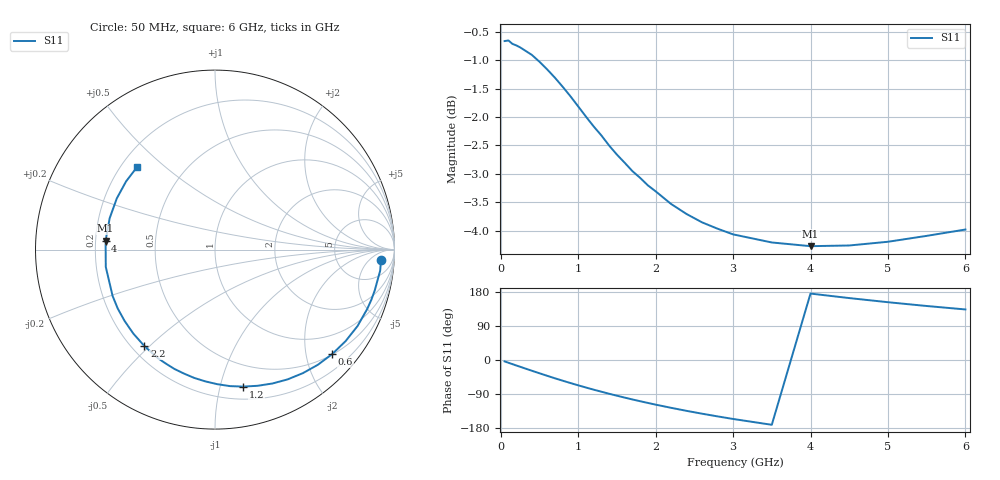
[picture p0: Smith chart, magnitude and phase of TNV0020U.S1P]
! SIEMENS Discrete & RF Semiconductors
! BAS70-07W
! Si Schottky Diode in SOT343
! IF = 0.02 mA
! S-Parameters:  February  1997
# GHz  S  MA  R  50
!  f  S11
! GHz  MAG  ANG
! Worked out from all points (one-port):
!   34 points, 50 MHz to 6 GHz, reference 50 ohm
!   lowest |S11| = -4.3 dB at 4 GHz (marker M1), VSWR 4.15, Z = 12.1 + j1.93 ohm
!   |S11| at or under -10 dB: nowhere
!   S11 on the Smith chart (normalised r, x): 50 MHz: 15, -13; 600 MHz: 0.51, -2.54; 1.2 GHz: 0.30, -1.18; 2.2 GHz: 0.25, -0.48; 4 GHz: 0.24, +0.04; 6 GHz: 0.26, +0.41
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0.05  0.9266 -3.7
0.1  0.9277 -7.3
0.15  0.9214 -10.8
0.3  0.9103 -21.3
0.4  0.9012 -28.2
0.5  0.8886 -35.0
0.6  0.8748 -41.7
0.7  0.8602 -48.3
0.8  0.8446 -54.6
0.9  0.8285 -60.8
1  0.8117 -66.8
1.2  0.7794 -78.3
1.4  0.7497 -89.1
1.6  0.7242 -99.2
1.8  0.7023 -108.8
1.9  0.6917 -113.3
2  0.6834 -117.8
2.2  0.6661 -126.2
2.4  0.6527 -134.2
2.6  0.6417 -141.7
2.8  0.6335 -148.8
3  0.6263 -155.6
3.5  0.6161 -171.0
4  0.6115 175.3
4.5  0.6124 163.4
5  0.617 152.5
5.5  0.6244 142.5
6  0.6325 133.4
